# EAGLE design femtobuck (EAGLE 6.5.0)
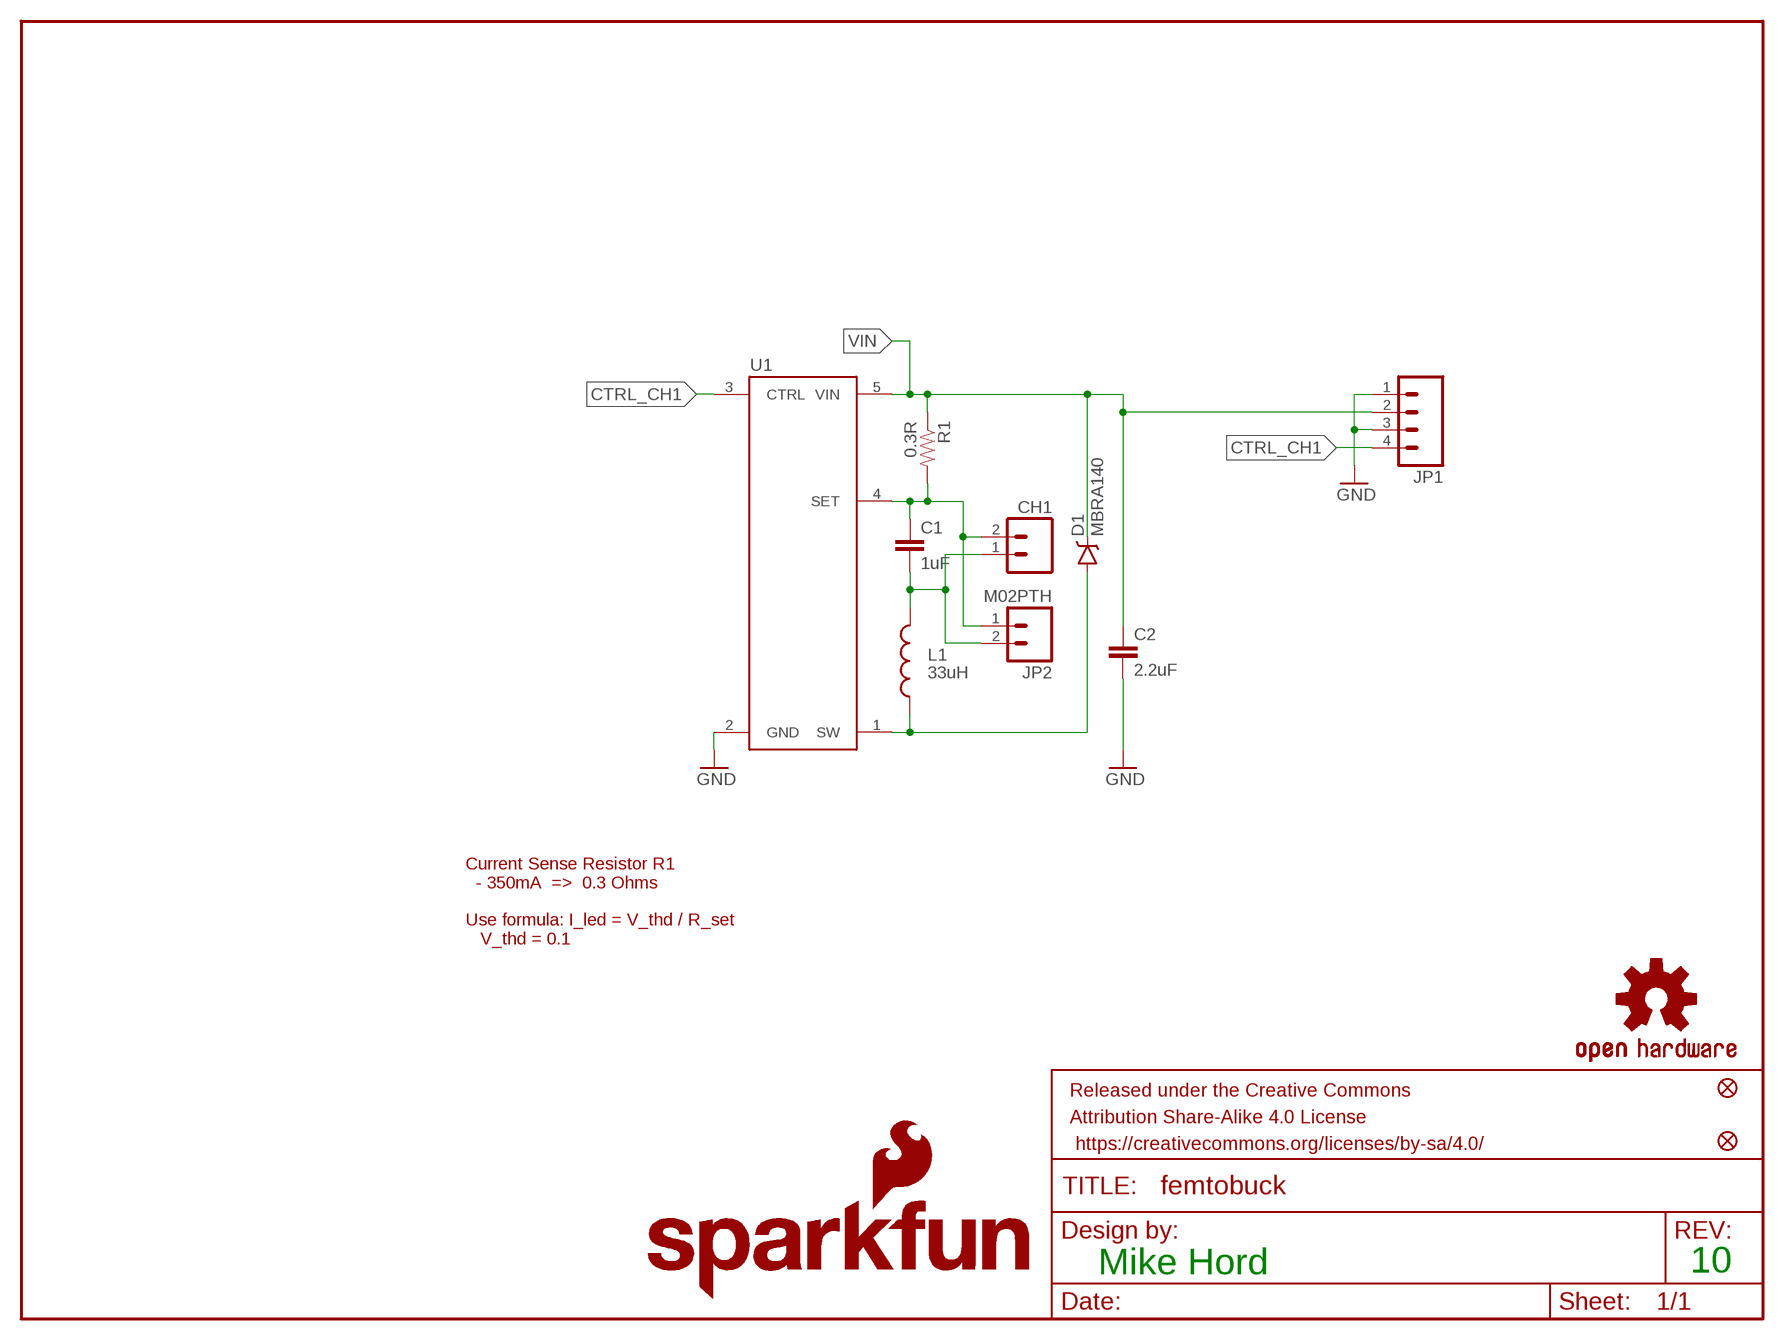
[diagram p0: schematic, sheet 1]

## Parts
C1  1uF  1.0UF50V10%(1206)  [1206]
C2  2.2uF  2.2UF50V10%(1206)  [1206]
CH1  M023.5MM_LOCK  [SCREWTERMINAL-3.5MM-2_LOCK]
D1  MBRA140  DIODE-SCHOTTKY-MBRA140  [SMA-DIODE]
FID1  FIDUCIAL1X2  [FIDUCIAL-1X2]
FID2  FIDUCIAL1X2  [FIDUCIAL-1X2]
FRAME1  FRAME-LETTER  [CREATIVE_COMMONS]
JP1  M04PTH  [1X04]
JP2  M02PTH  [1X02]
L1  33uH  INDUCTORBOURNS_SRN6045  [SRN6045]
LOGO1  OSHW-LOGOS  [OSHW-LOGO-S]
LOGO2  SFE_LOGO_NAME_FLAME.1_INCH  [SFE_LOGO_NAME_FLAME_.1]
R1  0.3R  0.3OHM-1/8W-1%(0805)  [0805]
U1  AL8805  [SOT23-5]

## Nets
CTRL_CH1: JP1.4 U1.3(CTRL)
GND: C2.2 JP1.1 JP1.3 U1.2(GND)
OUT+: C1.1 CH1.2 JP2.1 R1.2 U1.4(SET)
OUT- [power]: C1.2 CH1.1 JP2.2 L1.2
SW: D1.A L1.1 U1.1(SW)
VIN: C2.1 D1.C JP1.2 R1.1 U1.5(VIN)

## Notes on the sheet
- Current Sense Resistor R1
    - 350mA  =>  0.3 Ohms
  
  Use formula: I_led = V_thd / R_set
     V_thd = 0.1
- Mike Hord | 10

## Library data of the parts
C1 = SparkFun-Capacitors:1.0UF50V10%(1206): CAP-09822; PROD_ID: CAP-09822; VALUE: 1.0uF
C2 = SparkFun-Capacitors:2.2UF50V10%(1206): CAP-10009; PROD_ID: CAP-10009; VALUE: 2.2UF
CH1 = SparkFun:M02: Header 2
D1 = SparkFun-DiscreteSemi:DIODE-SCHOTTKY: Schottky diodes in SFE's production catalog; PROD_ID: DIO-08053
FID1 FID2 = SparkFun-Aesthetics:FIDUCIAL: Fiducial Alignment Points
FRAME1 = SparkFun-Aesthetics:FRAME-LETTER: Schematic Frame
JP1 = SparkFun-Connectors:M04: Header 4 Standard 4-pin 0.1" header. Use with straight break away headers (SKU : PRT-00116), right angle break away headers (PRT-00553), swiss pins (PRT-00743), machine pins (PRT-00117), and female headers (PRT-00115). Molex polarized connector foot print use with SKU : PRT-08231 with associated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
JP2 = SparkFun-Connectors:M02: Standard 2-pin 0.1" header. Use with
L1 = SparkFun-Passives:INDUCTOR: Inductors; PROD_ID: NDUC-11627
LOGO1 = SparkFun-Aesthetics:OSHW-LOGO: Open Source Hardware Logo This logo indicates the piece of hardware it is found on incorporates a OSHW license and/or adheres to the definition of open source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
LOGO2 = SparkFun-Aesthetics:SFE_LOGO_NAME_FLAME: SFE Logo, name and flame
R1 = SparkFun-Resistors:0.3OHM-1/8W-1%(0805): RES-11622; PROD_ID: RES-11622; VALUE: 0.3
U1 = SparkFun-PowerIC:AL8805: Constant current LED driver PWM-able 1MHz switch freq 6V-36V Up to 1A LED current; PROD_ID: IC-11626; VALUE: AL8805WS

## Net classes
0 default: width 0.254 mm
1 power: width 0.508 mm

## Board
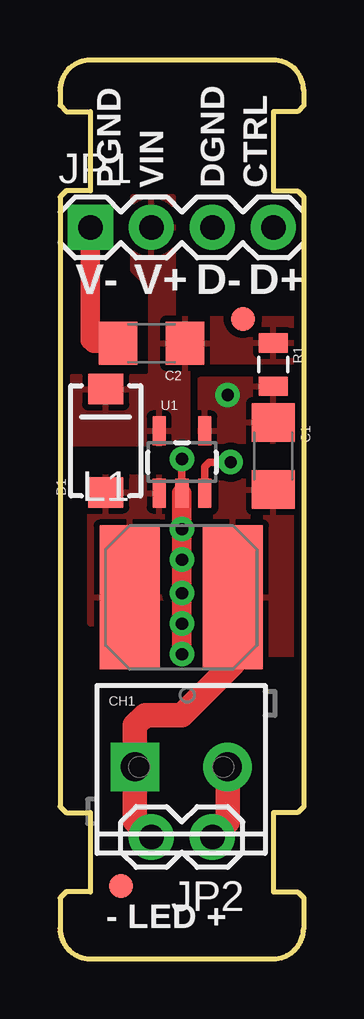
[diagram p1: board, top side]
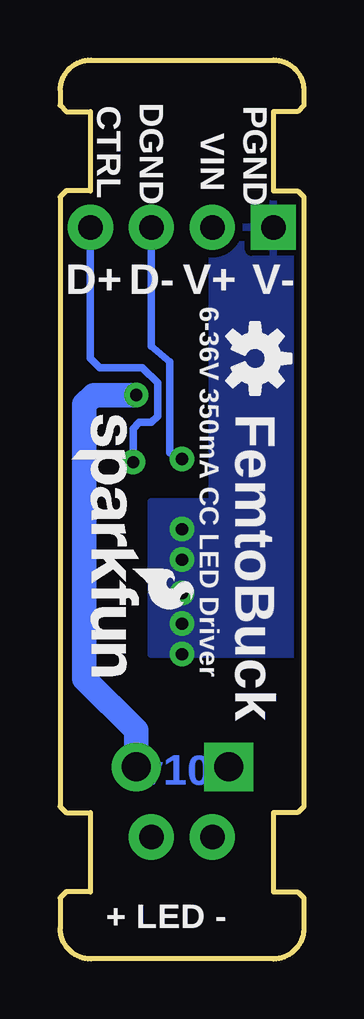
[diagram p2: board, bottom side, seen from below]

Size 10.16 x 37.45 mm. Coordinates in mm from the lower left corner, seen from the top.
Outline: 10.15,1.27 arc-90 8.88,0 1.27,0 arc-90 0,1.27 0,2.54 0.25,2.79 1.27,2.79 1.27,6.1 0.25,6.1 0,6.35 0,31.75 0.25,32 1.27,32 1.27,35.31 0.25,35.31 0,35.56 0,36.2
Outline: 10.15,36.18 arc90 8.88,37.45 1.27,37.45 arc90 0,36.18
Outline: 10.16,36.2 10.16,35.56 9.91,35.31 8.89,35.31 8.89,32 9.91,32 10.16,31.75 10.16,6.35 9.91,6.1 8.89,6.1 8.89,2.79 9.91,2.79 10.16,2.54 10.16,1.27
Copper layers (1*16): Top 0.035mm / dielectric 1.5mm / Bottom 0.035mm
Design rules "Sparkfun": minimum track width 8mil, minimum drill 20mil, track to track 8mil, track to pad 8mil, pad to pad 8mil, via to via 8mil, smd to smd 8mil, copper to edge 8mil, drill to drill 8mil, minimum pad ring 12mil, minimum via ring 10mil, stop-mask expansion 4mil, vias tented up to drill 20mil, thermal gap 10mil

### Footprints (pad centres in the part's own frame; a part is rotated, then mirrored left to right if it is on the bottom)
1206 = smd 1.6 x 1.8: 1 -1.4,0; 2 1.4,0
SCREWTERMINAL-3.5MM-2_LOCK = drill 1.2 pad 2.032 square: 1 -0.178,0 | drill 1.2 pad 2.032: 2 3.678,0
SMA-DIODE = smd 1.27 x 1.47: A -2.15,0; C 2.15,0
FIDUCIAL-1X2 = smd 1 x 1: 1 0,0
1X04 = drill 1.016 pad 1.88 square: 1 0,0 | drill 1.016 pad 1.88: 2 2.54,0; 3 5.08,0; 4 7.62,0
1X02 = drill 1.016 pad 1.88: 1 0,0; 2 2.54,0
SRN6045 = smd 2.5 x 6: 1 -2.175,-0.175; 2 2.125,-0.175
0805 = smd 0.8 x 1.2: 1 -0.9,0; 2 0.9,0
SOT23-5 = smd 0.55 x 1.2: 1 -0.95,-1.3; 2 0,-1.3; 3 0.95,-1.3; 4 0.95,1.3; 5 -0.95,1.3

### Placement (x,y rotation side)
C1  8.89,20.96 270 top
C2  3.81,25.65 180 top
CH1  3.3,8 0 top
D1  1.91,21.59 90 top
FID1  7.62,26.67 0 top
FID2  2.54,3.05 0 top
FRAME1  not placed on the board
JP1  1.27,30.48 0 top
JP2  6.35,5.08 180 top
L1  5.08,15.24 0 top
LOGO1  2.03,25.02 270 bottom
LOGO2  9.78,23.11 270 bottom
R1  8.89,24.77 270 top
U1  5.08,20.7 0 top

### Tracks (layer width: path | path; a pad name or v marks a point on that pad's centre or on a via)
CTRL_CH1  (via drill 0.51)
  Top 0.305: U1.3 6.03,20.51 6.22,20.7 v7.11,20.7
  Bottom 0.305: v7.11,20.7 7.11,22.1 6.86,22.35 6.35,22.35 6.1,22.61 6.1,24 6.73,24.64 8.51,24.64 8.89,25.02 JP1.4
GND  (via drill 0.51)
  Top 0.305: U1.2 v5.08,20.83
  Top 0.813: U1.2 v5.08,17.91 5.08,12.83 | JP1.1 1.27,25.78 1.4,25.65 C2.2
  Bottom 0.305: JP1.3 6.35,25.53 5.59,24.89 5.59,21.08 v5.08,20.83
  other vias: 5.08,16.64 5.08,15.24 5.08,13.97 5.08,12.7
  pour Bottom (isolate 0.305): 0,31.75 3.81,31.75 3.81,19.05 6.35,19.05 6.35,12.7 0,12.7
OUT+  (via drill 0.51)
  Top 1.016: CH1.2 6.98,5.71 JP2.1
  Bottom 1.016: v6.99,23.5 8.76,23.5 9.14,23.11 9.14,11.68 6.98,9.52 CH1.2
  pour Top (isolate 0.305): 8.89,24.13 5.84,24.13 5.84,21.59 8.89,21.59
OUT-
  Top 1.016: L1.2 7.21,12.29 5.08,10.16 3.56,10.16 3.12,9.73 CH1.1 3.12,5.77 JP2.2
  pour Top (isolate 0.305): 6.35,20.07 10.16,20.07 10.16,12.7 6.35,12.7
SW
  pour Top (isolate 0.305): 1.27,20.07 5.08,20.07 5.08,13.97 1.27,13.97
VIN
  pour Top (isolate 0.305, rank 2): 3.05,31.75 4.7,31.75 4.7,26.8 4.83,26.67 9.78,26.67 9.78,24.89 6.22,24.89 5.59,24.26 5.59,21.46 0.51,21.46 0.51,24.26 3.68,24.26 3.81,24.38 3.81,27.94 3.05,28.7

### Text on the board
Bottom: v10
tPlace: PGND | VIN | DGND | CTRL | V- | V+ | D- | D+ | - LED +
bPlace: PGND | DGND | CTRL | VIN | V- | V+ | D- | D+ | 6-36V 350mA CC LED Driver | FemtoBuck | + LED -
tDocu: M. Hord

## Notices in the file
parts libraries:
SparkFun-Aesthetics: Licensing: CC v3.0 Share-Alike You are welcome to use this library for commercial purposes.
SparkFun-Aesthetics: Released under the Creative Commons Attribution Share-Alike 4.0 License
SparkFun-Aesthetics: https://creativecommons.org/licenses/by-sa/4.0
